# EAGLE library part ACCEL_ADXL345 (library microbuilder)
ADXL345 - Digital 3-Axis Accelerometer (I2C/SPI)
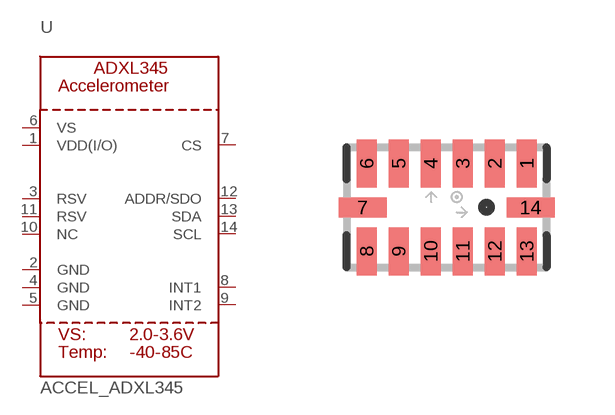
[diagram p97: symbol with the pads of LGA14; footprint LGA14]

Designator prefix U

## ACCEL_ADXL345  [LGA14]
1  VDD(I/O)
2  GND
3  RSV
4  GND
5  GND
6  VS
7  CS
8  INT1
9  INT2
10  NC
11  RSV
12  ADDR/SDO
13  SDA
14  SCL

## Footprint LGA14 (pad centres in mm)
smd 0.5 x 1.2: 1 2,1.1; 2 1.2,1.1; 3 0.4,1.1; 4 -0.4,1.1; 5 -1.2,1.1; 6 -2,1.1; 8 -2,-1.1; 9 -1.2,-1.1; 10 -0.4,-1.1; 11 0.4,-1.1; 12 1.2,-1.1; 13 2,-1.1
smd 1.2 x 0.5: 7 -2.1,0; 14 2.1,0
